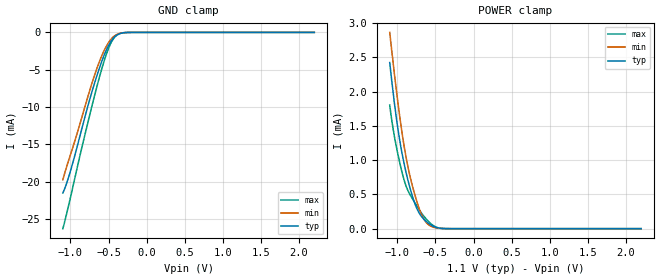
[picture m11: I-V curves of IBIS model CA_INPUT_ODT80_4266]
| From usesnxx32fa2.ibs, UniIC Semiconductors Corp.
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| CA_INPUT_ODT80_4266 (with 80ohm ODT, 3200-4266Mbps)
[Model]   CA_INPUT_ODT80_4266
Model_type   Input
Vinl = 110.833mV
Vinh = 255.833mV
|   typ   min   max
|C_comp   0.664pF   0.616pF   0.719pF
C_comp_power_clamp   0.3320pF   0.3080pF   0.3595pF
C_comp_gnd_clamp   0.3320pF   0.3080pF   0.3595pF
| Note: C_comp changes when the ODT circuit is enabled.
[Model Spec]
| Input threshold voltage corners
Vinl   0.1108V   0.1042V   0.1225V
Vinh   0.2558V   0.2492V   0.2675V
| Dynamic Overshoot Parameters from LPDDR4 Specification
D_overshoot_ampl_h   0.30   NA   NA
D_overshoot_ampl_l   0.30   NA   NA
D_overshoot_area_h   0.1n   NA   NA
D_overshoot_area_l   0.1n   NA   NA
[Voltage Range]   1.1000V   1.0600V   1.1700V
[POWER Clamp Reference]   1.1000V   1.0600V   1.1700V
| Junction Temperature (Ambient temp is 35C typ 95C min -40C max)
[Temperature Range]   50.0   110.0   -40.0
[Add Submodel]
| Submodel Name   Mode
80ohm_ODT_4266   Non-Driving
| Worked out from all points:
|   GND clamp passes 1 mA (typ) near -0.45 V on its own axis
|   POWER clamp passes 1 mA (typ) near -0.92 V on its own axis
[GND Clamp]
|   Voltage   I(typ)   I(min)   I(max)
-1.1V     -21.5mA    -19.73mA   -26.28mA
-1.057V   -20.41mA   -18.22mA   -24.57mA
-1.001V   -18.6mA    -16.41mA   -22.15mA
-763.4mV  -9.562mA   -8.321mA   -11.73mA
-680.9mV  -6.696mA   -5.635mA   -8.352mA
-614.9mV  -4.625mA   -3.777mA   -5.81mA
-552.2mV  -2.909mA   -2.311mA   -3.642mA
-496.1mV  -1.68mA    -1.302mA   -2.041mA
-446.6mV  -895.5uA   -681.9uA   -1.019mA
-397.1mV  -403uA     -305.7uA   -413.1uA
-248.6mV  -11.98uA   -10.81uA   -7.088uA
2.2V      0A         0A         0A
[POWER Clamp]
|   Voltage   I(typ)   I(min)   I(max)
-1.1V     2.422mA    2.862mA    1.802mA
-1.041V   1.851mA    2.277mA    1.359mA
-981.2mV  1.374mA    1.741mA    1.027mA
-921.8mV  1.005mA    1.277mA    751.6uA
-862.4mV  713uA      909uA      559.1uA
-783.2mV  406.3uA    545.8uA    401.7uA
-710.6mV  222.9uA    283.8uA    272.7uA
-657.8mV  145uA      149.1uA    190.3uA
-588.5mV  74.68uA    55.78uA    101.5uA
-496.1mV  19.98uA    11.76uA    25.38uA
-370.7mV  1.131uA    772.7nA    812.6nA
2.2V      0A         0A         0A
